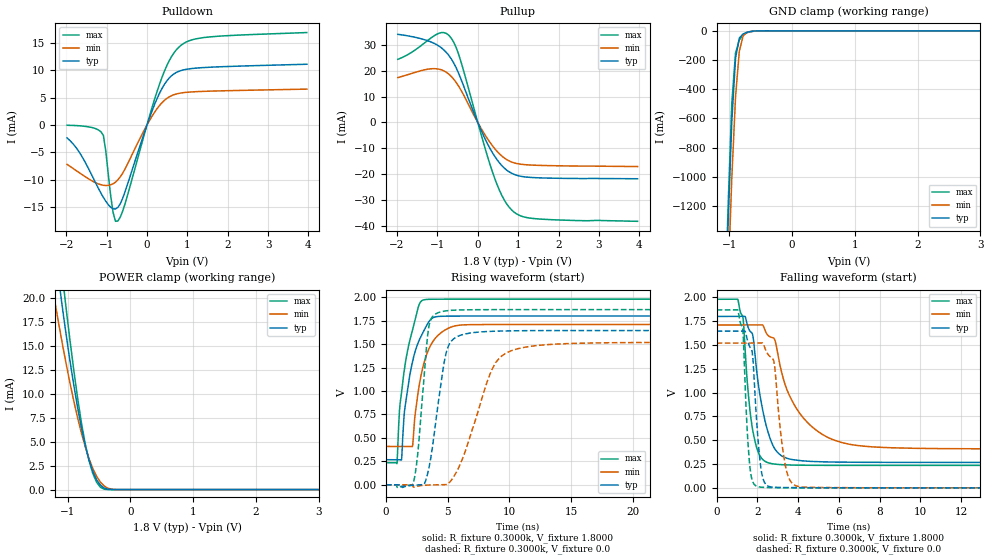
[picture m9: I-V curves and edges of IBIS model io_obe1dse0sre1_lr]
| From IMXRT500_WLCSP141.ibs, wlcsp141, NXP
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[Model] io_obe1dse0sre1_lr
|   Model io_obe1dse0sre1_lr
| Library cells for typ/min/max conditions are connected as defined below:
|  pad - External Pad
|  ipp_do - Core Input
|  ipp_obe - Output Buffer Enable
|  REFH3V3 - vdd1v8
|  gnde - gnde
|  ipp_ina235_3v - NC
|  ipp_ina40_3v - NC
|  ipp_ina_mux - NC
|  ipp_ind - NC
|  ipp_ind_1p8v - NC
|  ipp_ind_3v - NC
|  ipp_sre - vdd
|  vdd - vdd
|  vdd1v8 - vdd1v8
|  vdda - vdde3v3
|  vdde3v3 - vdde3v3
| All other pins connected to ground
Model_type I/O
Polarity   Non-Inverting
Enable   Active-High
Vinl =   0.5400V
Vinh =   1.2600V
Vmeas =  0.9000V
Cref =   25.0000pF
Rref =   0.5000k
Vref =   0.0V
C_comp   2.2672pF   2.1739pF   2.3940pF
[Temperature Range]   25.0000   0.1250k   -40.0000
[Voltage Range]   1.8000V   1.7100V   1.9800V
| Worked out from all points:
|   slope of the pulldown table from 0 to 0.27 V, typ, clamps not added: 52.5 ohm
|   slope of the pullup table from 0 to 0.27 V, typ, clamps not added: 29.8 ohm
|   GND clamp passes 1 mA (typ) near -0.57 V on its own axis
|   POWER clamp passes 1 mA (typ) near -0.54 V on its own axis
|   rising waveform, R_fixture 0.3000k, V_fixture 1.8000: 20-80 % time 1.16ns typ, 1.18ns min, 1.1ns max; typ from 0.267 V to 1.8 V
|   rising waveform, R_fixture 0.3000k, V_fixture 0.0: 20-80 % time 1.05ns typ, 2.26ns min, 693ps max; typ from 0 V to 1.65 V
|   falling waveform, R_fixture 0.3000k, V_fixture 1.8000: 20-80 % time 700ps typ, 1.58ns min, 439ps max; typ from 1.8 V to 0.267 V
|   falling waveform, R_fixture 0.3000k, V_fixture 0.0: 20-80 % time 312ps typ, 440ps min, 244ps max; typ from 1.65 V to 0 V
[Pulldown]
|Voltage   I(typ)   I(min)   I(max)
-1.98V    -2.37mA    -7.2mA     -50uA
-1.62V    -5.66mA    -9.02mA    -180uA
-1.08V    -13.25mA   -11.03mA   -1.913mA
-840mV    -15.32mA   -10.75mA   -15.99mA
-780mV    -15.35mA   -10.45mA   -17.61mA
-720mV    -15.07mA   -10.02mA   -17.56mA
-540mV    -12.12mA   -7.995mA   -14.33mA
240mV     4.654mA    2.876mA    5.906mA
540mV     8.495mA    5.085mA    11.58mA
780mV     9.772mA    5.756mA    14.15mA
1.44V     10.5mA     6.149mA    16mA
3.96V     11.1mA     6.548mA    16.88mA
[Pullup]
|Voltage   I(typ)   I(min)   I(max)
-1.98V    34mA       17.32mA    24.37mA
-960mV    29.45mA    20.56mA    34.44mA
-780mV    27.06mA    19.38mA    34.35mA
-660mV    24.61mA    17.81mA    32.59mA
-540mV    21.23mA    15.54mA    29.04mA
-420mV    16.88mA    12.58mA    23.61mA
60mV      -2.204mA   -1.665mA   -3.362mA
420mV     -13.07mA   -10.1mA    -21.6mA
660mV     -17.64mA   -13.73mA   -30.01mA
960mV     -20.35mA   -15.82mA   -35.25mA
1.62V     -21.4mA    -16.59mA   -37.33mA
3.96V     -21.71mA   -17.01mA   -38.12mA
[GND_clamp]
|Voltage   I(typ)   I(min)   I(max)
-1.98V    -17.54A    -17.55A    -18.13A
-1.08V    -2.178A    -2.567A    -2.121A
-1.02V    -1.334A    -1.74A     -1.223A
-960mV    -626.1mA   -1.012A    -499.4mA
-900mV    -186.7mA   -452.2mA   -152mA
-840mV    -49.63mA   -139.9mA   -62.86mA
-780mV    -21.48mA   -35.54mA   -26.58mA
-720mV    -10.4mA    -11.15mA   -13.18mA
-600mV    -1.573mA   -2.152mA   -2.249mA
-480mV    -123.2uA   -243.9uA   -63.17uA
3.96V     0A         0A         0A
[POWER_clamp]
|Voltage   I(typ)   I(min)   I(max)
-1.98V    72.06mA    51.35mA    77.71mA
-1.26V    28.12mA    21.78mA    33.04mA
-1.2V     24.9mA     19.47mA    29.3mA
-1.14V    21.8mA     17.23mA    25.64mA
-1.08V    18.82mA    15.06mA    22.09mA
-1.02V    15.98mA    12.99mA    18.67mA
-840mV    8.51mA     7.462mA    9.493mA
-720mV    4.608mA    4.475mA    4.783mA
-600mV    1.908mA    2.218mA    1.702mA
-540mV    1.04mA     1.402mA    786.7uA
-420mV    173.6uA    383.7uA    43.39uA
3.96V     0A         0A         0A
[Ramp]
| variable   typ   min   max
dV/dt_r  0.5846/2.4351n   0.4707/4.8778n   0.8358/1.3679n
dV/dt_f  0.3128/1.5333n   0.1842/2.5261n   0.4711/1.0699n
R_load = 50.0000
[Rising Waveform]
R_fixture= 0.3000k
V_fixture= 1.8000
V_fixture_min= 1.7100
V_fixture_max= 1.9800
|time   V(typ)   V(min)   V(max)
0s        267.3mV    408.9mV    235.9mV
898.7ps   267.3mV    408.9mV    227.4mV
1.092ns   267.3mV    408.9mV    769.8mV
1.267ns   267.2mV    408.9mV    981.1mV
1.522ns   799.2mV    408.9mV    1.25V
2.151ns   1.309V     410.3mV    1.645V
2.73ns    1.551V     1.082V     1.932V
3.577ns   1.755V     1.474V     1.978V
8.133ns   1.8V       1.709V     1.98V
500ns     1.8V       1.71V      1.98V
[Rising Waveform]
R_fixture= 0.3000k
V_fixture= 0.0
V_fixture_min= 0.0
V_fixture_max= 0.0
|time   V(typ)   V(min)   V(max)
0s        30.08nV    1.925uV    117.4nV
2.213ns   -5.544mV   -21.68mV   16.33mV
2.582ns   -2.68mV    -14.19mV   328.6mV
3.144ns   16.23mV    -5.261mV   1.234V
3.595ns   252mV      -2.461mV   1.747V
4.854ns   1.389V     1.625mV    1.855V
5.989ns   1.592V     208.1mV    1.865V
9.289ns   1.64V      1.364V     1.868V
16.68ns   1.645V     1.512V     1.868V
500ns     1.645V     1.52V      1.868V
[Falling Waveform]
R_fixture= 0.3000k
V_fixture= 1.8000
V_fixture_min= 1.7100
V_fixture_max= 1.9800
|time   V(typ)   V(min)   V(max)
0s        1.8V       1.71V      1.98V
1.032ns   1.8V       1.71V      1.981V
1.276ns   1.799V     1.71V      1.802V
1.658ns   1.641V     1.71V      770.4mV
2.078ns   1.037V     1.709V     355.1mV
2.785ns   435.7mV    1.574V     251.5mV
3.869ns   291.5mV    850.7mV    238.5mV
6.162ns   269.9mV    475mV      236.1mV
11.88ns   267.4mV    410.9mV    236mV
500ns     267.3mV    408.9mV    235.9mV
[Falling Waveform]
R_fixture= 0.3000k
V_fixture= 0.0
V_fixture_min= 0.0
V_fixture_max= 0.0
|time   V(typ)   V(min)   V(max)
0s        1.645V     1.52V      1.868V
1.045ns   1.645V     1.52V      1.865V
1.286ns   1.645V     1.52V      1.648V
1.413ns   1.637V     1.52V      987.2mV
1.737ns   1.434V     1.52V      84.83mV
2.192ns   178.6mV    1.522V     6.824mV
2.806ns   6.661mV    1.332V     2.029mV
3.524ns   2.996mV    114.1mV    634.7uV
5.258ns   733uV      3.37mV     71.77uV
500ns     1.047uV    3.184uV    785.2nV
